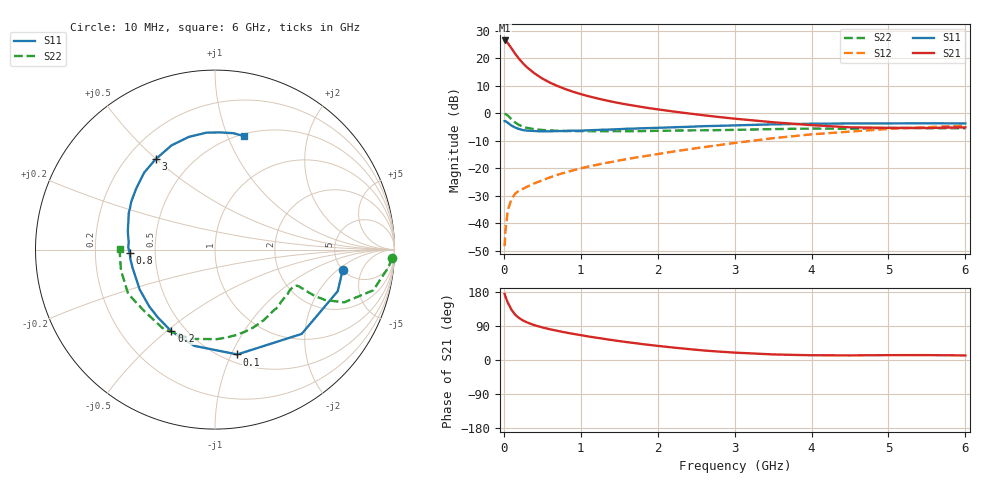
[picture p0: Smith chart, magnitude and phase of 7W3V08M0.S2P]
! Infineon Technologies  Discrete & RF Semiconductors
! BFS17W
! Si NPN RF Bipolar Junction Transistor in SOT323
! VCE = 3 V  IC = 8 mA
! Common Emitter S-Parameters:  August  1999
# GHz  S  MA  R  50
!  f  S11  S21  S12  S22
! GHz  MAG  ANG  MAG  ANG  MAG  ANG  MAG  ANG
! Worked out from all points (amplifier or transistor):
!   36 points, 10 MHz to 6 GHz, reference 50 ohm
!   highest |S21| = 26.5 dB at 10 MHz (marker M1)
!   |S21| within 3 dB of that: start of sweep to 102.6 MHz
!   unconditionally stable (mu >= 1): 437.9 MHz to 2.641 GHz; 4.341 GHz to end of sweep
!   at 250 MHz: K = 0.74, MSG = 22.8 dB, |S12| = -27.5 dB
!   at 1.4 GHz: K = 1.23, MAG = 8.1 dB, |S12| = -17.7 dB
!   at 6 GHz: K = 1.07, MAG = -2.0 dB, |S12| = -4.5 dB
!   S11 on the Smith chart (normalised r, x): 10 MHz: 4.97, -2.38; 100 MHz: 0.58, -1.05; 200 MHz: 0.42, -0.52; 800 MHz: 0.36, -0.02; 3 GHz: 0.31, +0.50; 6 GHz: 0.52, +1.14
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0.01  0.7202 -9.2  21.21 174.5  0.0038 84.9  0.9899 -2.7
0.02  0.7221 -18.7  21.03 168.1  0.007 83.0  0.967 -6.3
0.05  0.6737 -44.2  19.16 152.0  0.0169 71.3  0.9108 -14.4
0.1  0.5971 -78.0  15.2 132.3  0.0277 58.4  0.7775 -22.2
0.15  0.5485 -102.2  12 119.1  0.0346 52.5  0.6745 -24.6
0.2  0.5161 -118.1  9.733 110.5  0.0391 52.6  0.6105 -24.9
0.25  0.4941 -130.2  8.085 104.2  0.0422 51.4  0.5686 -24.5
0.3  0.4843 -139.2  6.895 99.3  0.0458 52.5  0.5437 -24.1
0.4  0.4749 -152.1  5.312 91.7  0.0533 54.5  0.5118 -23.7
0.5  0.4681 -161.0  4.304 86.0  0.0601 56.6  0.4972 -23.8
0.6  0.4703 -167.6  3.611 81.1  0.0681 58.9  0.4871 -24.6
0.8  0.4759 -177.7  2.76 72.7  0.0837 61.8  0.4764 -27.7
0.9  0.4834 178.4  2.465 69.1  0.0914 62.5  0.473 -29.4
1.1  0.49 171.0  2.046 62.0  0.1072 63.6  0.4715 -33.8
1.3  0.5025 164.5  1.753 55.8  0.1232 64.6  0.4696 -38.7
1.6  0.5226 156.7  1.445 47.2  0.1464 65.8  0.4708 -46.4
2.2  0.5558 142.0  1.08 32.9  0.2004 66.6  0.4833 -63.9
3  0.6022 123.4  0.798 19.5  0.2881 63.8  0.4991 -88.7
3.5  0.6291 112.7  0.687 14.7  0.3519 59.8  0.5153 -105.1
4.5  0.6535 94.1  0.555 12.2  0.464 47.5  0.522 -138.7
5.5  0.6566 80.9  0.54 12.9  0.5589 35.0  0.5363 -167.8
6  0.6528 75.8  0.555 12.1  0.5957 28.9  0.532 179.5
